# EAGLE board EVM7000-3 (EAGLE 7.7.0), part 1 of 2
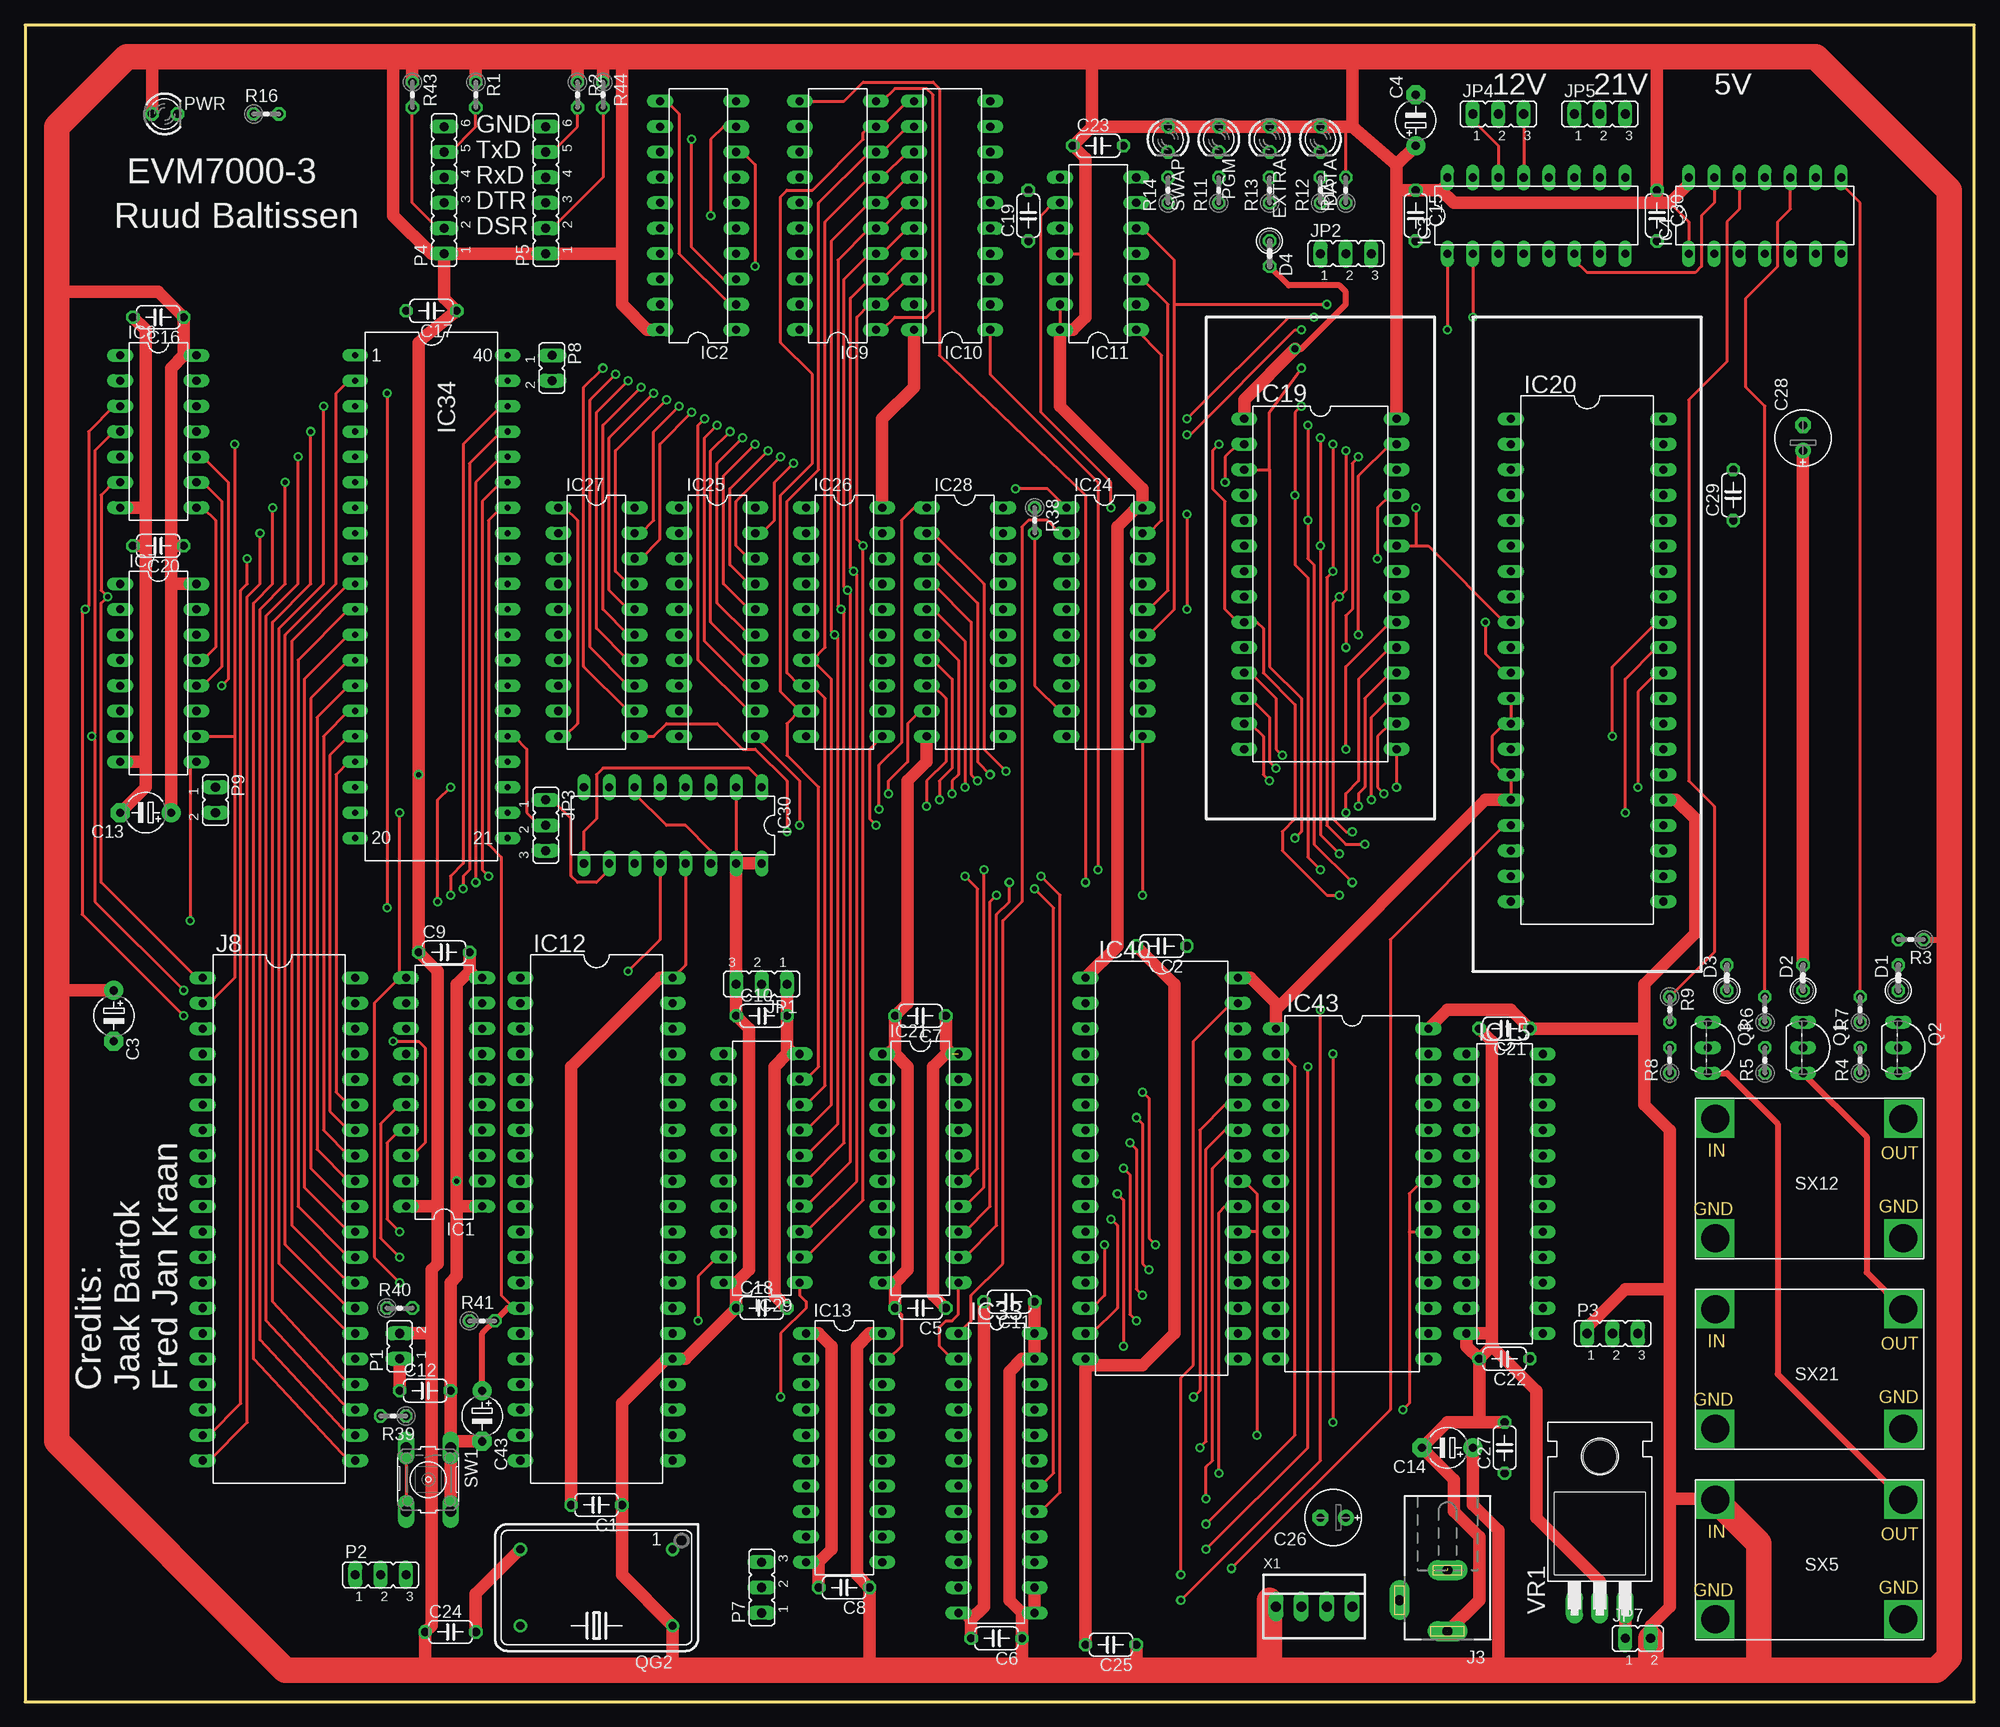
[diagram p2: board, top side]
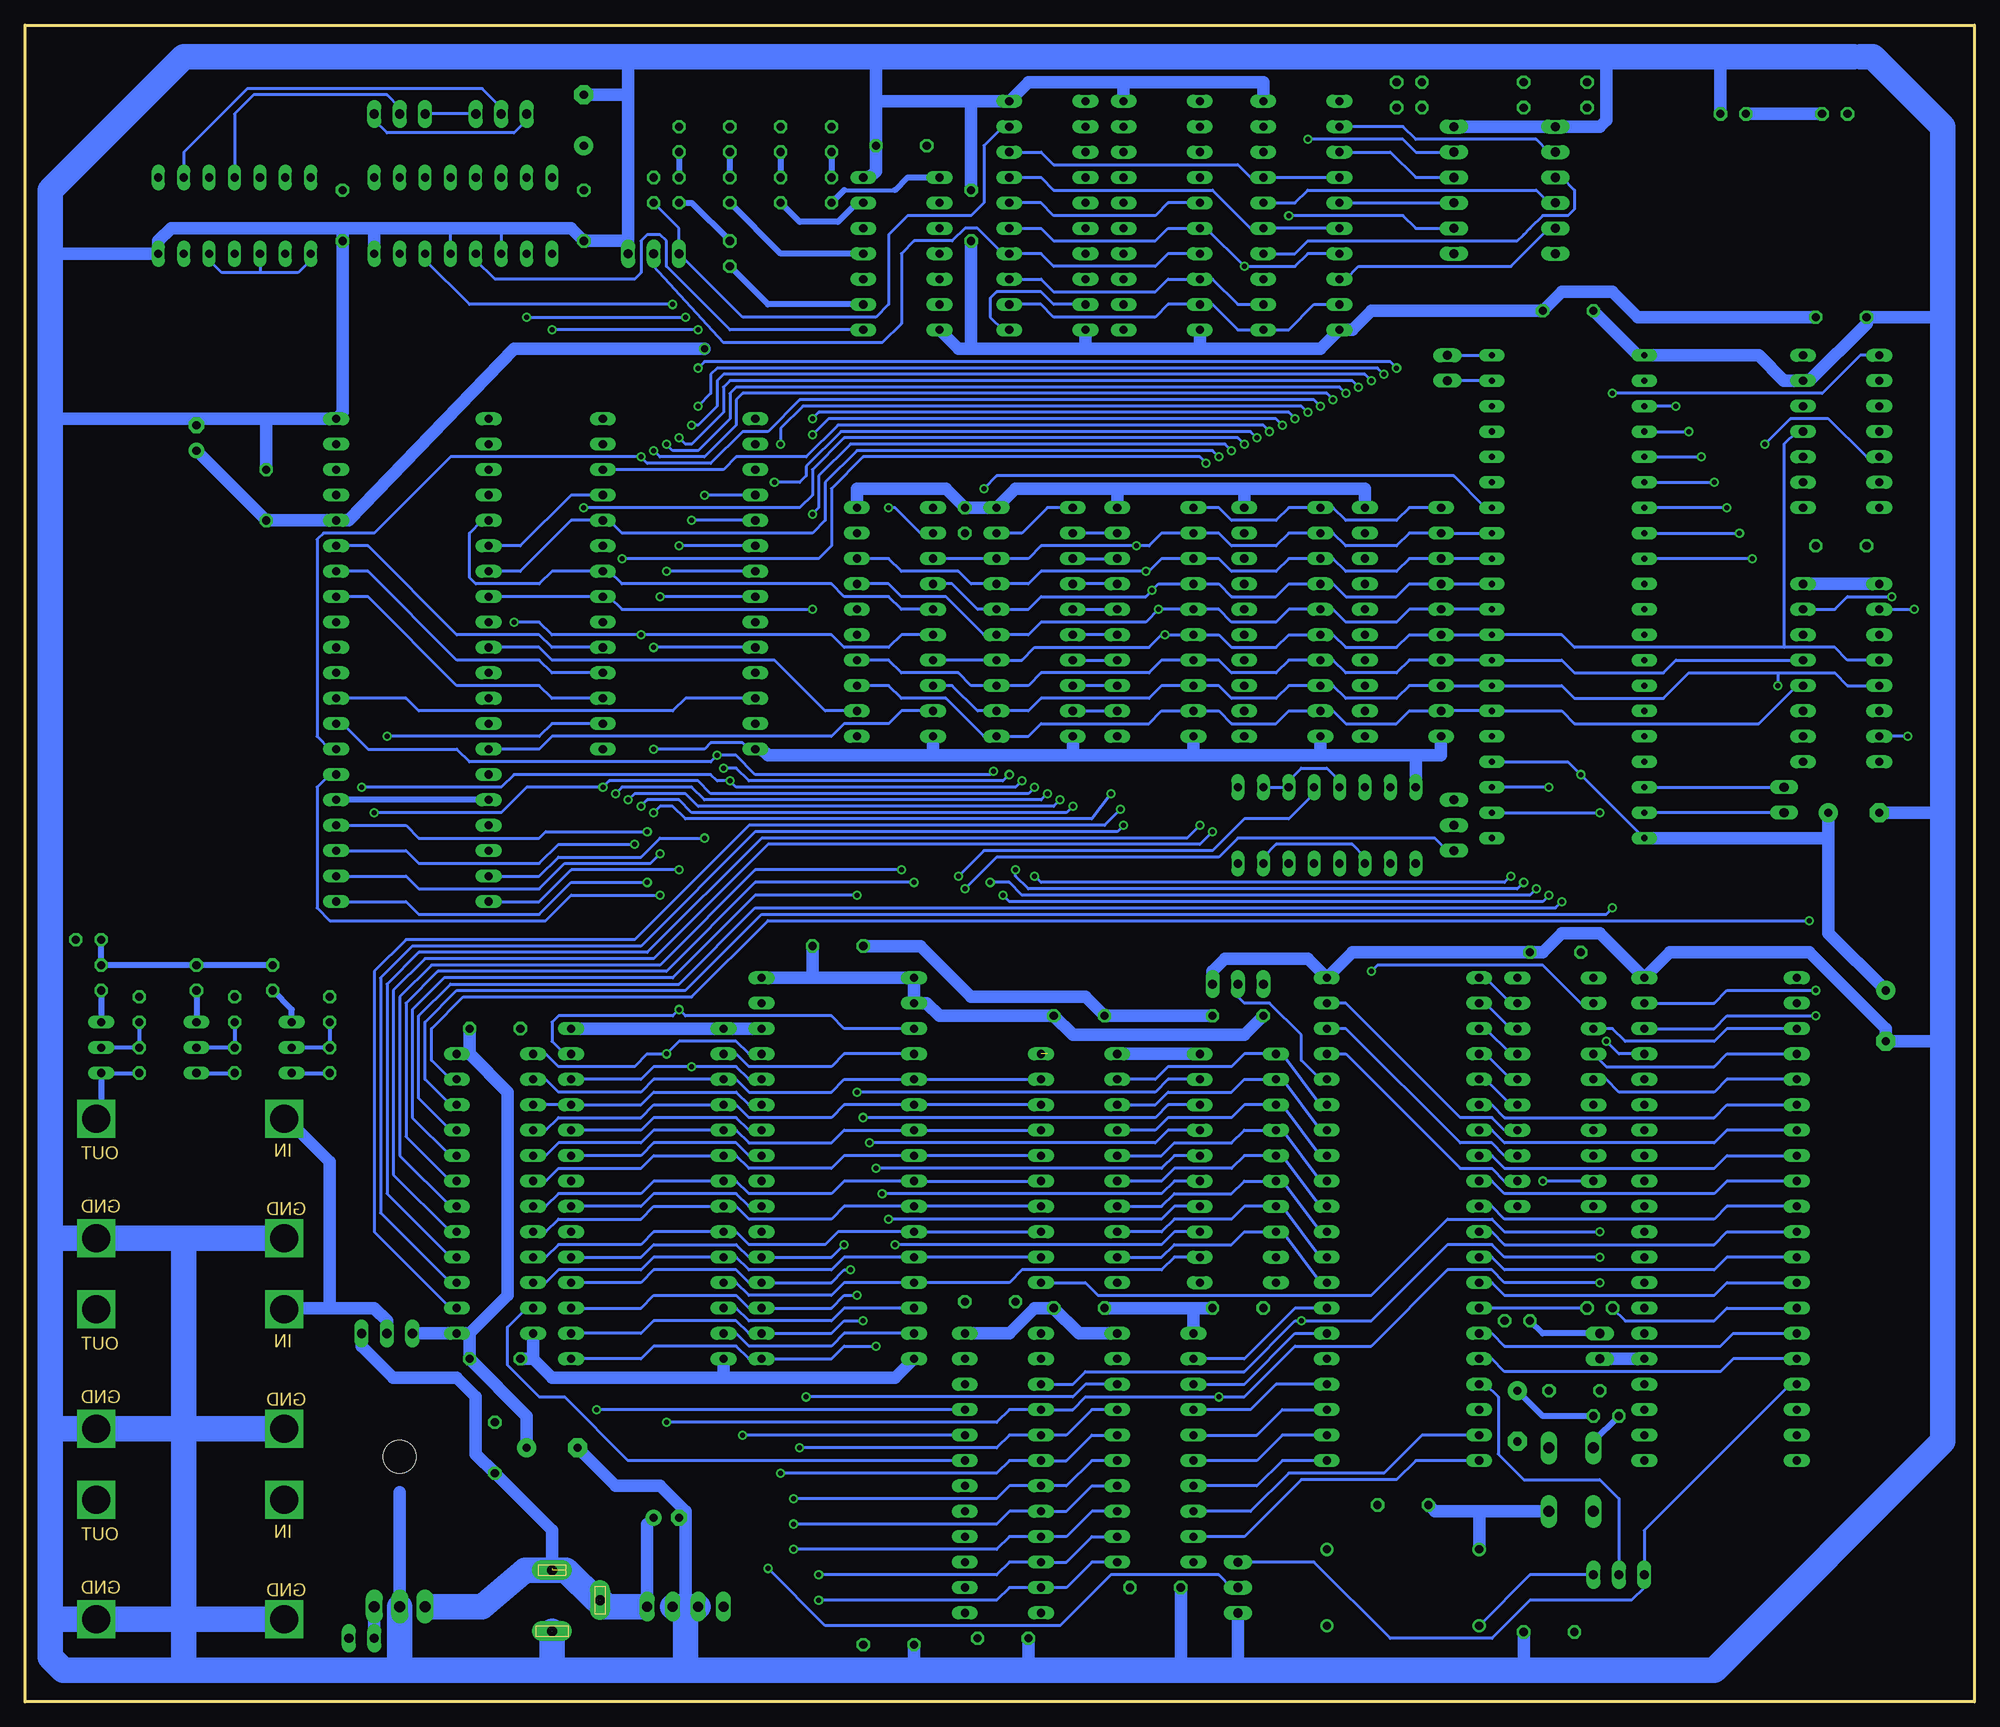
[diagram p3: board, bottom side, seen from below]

Size 194.94 x 167.64 mm. Coordinates in mm from the lower left corner, seen from the top.
Outline: 0,0 194.94,0 194.94,167.64 0,167.64 0,0
Copper layers (1*16): Top 0.035mm / dielectric 1.5mm / Bottom 0.035mm
Design rules "default": minimum track width 10mil, minimum drill 24mil, track to track 8mil, track to pad 8mil, pad to pad 8mil, via to via 8mil, smd to smd 8mil, copper to edge 40mil, drill to drill 8mil, minimum pad ring 10mil, minimum via ring 8mil, stop-mask expansion 4mil, vias tented up to drill 0mil, thermal gap 10mil

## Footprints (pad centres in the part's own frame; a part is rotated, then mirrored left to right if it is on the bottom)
C050-024X044 = drill 0.813 octagon: 1 -2.54,0; 2 2.54,0
E5-4 = drill 0.813 pad 1.905: + -2.54,0 | drill 0.813 pad 1.905 octagon: - 2.54,0
E2,5-6E = drill 0.813 pad 1.575: + -1.27,0 | drill 0.813 pad 1.575 octagon: - 1.27,0
0207/2V = drill 0.813 octagon: 1 -1.27,0; 2 1.27,0
LED3MM = drill 0.813 octagon: A -1.27,0; K 1.27,0
DIL20 = drill 0.813 long: 1 -11.43,-3.81; 2 -8.89,-3.81; 3 -6.35,-3.81; 4 -3.81,-3.81; 5 -1.27,-3.81; 6 1.27,-3.81; 7 3.81,-3.81; 8 6.35,-3.81; 9 8.89,-3.81; 10 11.43,-3.81; 11 11.43,3.81; 12 8.89,3.81; 13 6.35,3.81; 14 3.81,3.81; 15 1.27,3.81; 16 -1.27,3.81; 17 -3.81,3.81; 18 -6.35,3.81; 19 -8.89,3.81; 20 -11.43,3.81
DIL16 = drill 0.813 long: 1 -8.89,-3.81; 2 -6.35,-3.81; 3 -3.81,-3.81; 4 -1.27,-3.81; 5 1.27,-3.81; 6 3.81,-3.81; 7 6.35,-3.81; 8 8.89,-3.81; 9 8.89,3.81; 10 6.35,3.81; 11 3.81,3.81; 12 1.27,3.81; 13 -1.27,3.81; 14 -3.81,3.81; 15 -6.35,3.81; 16 -8.89,3.81
DIL14 = drill 0.813 long: 1 -7.62,-3.81; 2 -5.08,-3.81; 3 -2.54,-3.81; 4 0,-3.81; 5 2.54,-3.81; 6 5.08,-3.81; 7 7.62,-3.81; 8 7.62,3.81; 9 5.08,3.81; 10 2.54,3.81; 11 0,3.81; 12 -2.54,3.81; 13 -5.08,3.81; 14 -7.62,3.81
DIL40 = drill 0.813 long: 1 -24.13,-7.62; 2 -21.59,-7.62; 3 -19.05,-7.62; 4 -16.51,-7.62; 5 -13.97,-7.62; 6 -11.43,-7.62; 7 -8.89,-7.62; 8 -6.35,-7.62; 9 -3.81,-7.62; 10 -1.27,-7.62; 11 1.27,-7.62; 12 3.81,-7.62; 13 6.35,-7.62; 14 8.89,-7.62; 15 11.43,-7.62; 16 13.97,-7.62; 17 16.51,-7.62; 18 19.05,-7.62; 19 21.59,-7.62; 20 24.13,-7.62; 21 24.13,7.62; 22 21.59,7.62; 23 19.05,7.62; 24 16.51,7.62; 25 13.97,7.62; 26 11.43,7.62; 27 8.89,7.62; 28 6.35,7.62; 29 3.81,7.62; 30 1.27,7.62; 31 -1.27,7.62; 32 -3.81,7.62; 33 -6.35,7.62; 34 -8.89,7.62; 35 -11.43,7.62; 36 -13.97,7.62; 37 -16.51,7.62; 38 -19.05,7.62; 39 -21.59,7.62; 40 -24.13,7.62
DIL24-3 = drill 0.813 long: 1 -13.97,-3.81; 2 -11.43,-3.81; 3 -8.89,-3.81; 4 -6.35,-3.81; 5 -3.81,-3.81; 6 -1.27,-3.81; 7 1.27,-3.81; 8 3.81,-3.81; 9 6.35,-3.81; 10 8.89,-3.81; 11 11.43,-3.81; 12 13.97,-3.81; 13 13.97,3.81; 14 11.43,3.81; 15 8.89,3.81; 16 6.35,3.81; 17 3.81,3.81; 18 1.27,3.81; 19 -1.27,3.81; 20 -3.81,3.81; 21 -6.35,3.81; 22 -8.89,3.81; 23 -11.43,3.81; 24 -13.97,3.81
DIL28 = drill 0.813 long: 1 -16.51,-7.62; 2 -13.97,-7.62; 3 -11.43,-7.62; 4 -8.89,-7.62; 5 -6.35,-7.62; 6 -3.81,-7.62; 7 -1.27,-7.62; 8 1.27,-7.62; 9 3.81,-7.62; 10 6.35,-7.62; 11 8.89,-7.62; 12 11.43,-7.62; 13 13.97,-7.62; 14 16.51,-7.62; 15 16.51,7.62; 16 13.97,7.62; 17 11.43,7.62; 18 8.89,7.62; 19 6.35,7.62; 20 3.81,7.62; 21 1.27,7.62; 22 -1.27,7.62; 23 -3.81,7.62; 24 -6.35,7.62; 25 -8.89,7.62; 26 -11.43,7.62; 27 -13.97,7.62; 28 -16.51,7.62
DIP40 = drill 0.61 pad 1.27 long: 1 -24.13,-7.62; 2 -21.59,-7.62; 3 -19.05,-7.62; 4 -16.51,-7.62; 5 -13.97,-7.62; 6 -11.43,-7.62; 7 -8.89,-7.62; 8 -6.35,-7.62; 9 -3.81,-7.62; 10 -1.27,-7.62; 11 1.27,-7.62; 12 3.81,-7.62; 13 6.35,-7.62; 14 8.89,-7.62; 15 11.43,-7.62; 16 13.97,-7.62; 17 16.51,-7.62; 18 19.05,-7.62; 19 21.59,-7.62; 20 24.13,-7.62; 21 24.13,7.62; 22 21.59,7.62; 23 19.05,7.62; 24 16.51,7.62; 25 13.97,7.62; 26 11.43,7.62; 27 8.89,7.62; 28 6.35,7.62; 29 3.81,7.62; 30 1.27,7.62; 31 -1.27,7.62; 32 -3.81,7.62; 33 -6.35,7.62; 34 -8.89,7.62; 35 -11.43,7.62; 36 -13.97,7.62; 37 -16.51,7.62; 38 -19.05,7.62; 39 -21.59,7.62; 40 -24.13,7.62
DIL32-6 = drill 0.813 long: 1 -19.05,-7.62; 2 -16.51,-7.62; 3 -13.97,-7.62; 4 -11.43,-7.62; 5 -8.89,-7.62; 6 -6.35,-7.62; 7 -3.81,-7.62; 8 -1.27,-7.62; 9 1.27,-7.62; 10 3.81,-7.62; 11 6.35,-7.62; 12 8.89,-7.62; 13 11.43,-7.62; 14 13.97,-7.62; 15 16.51,-7.62; 16 19.05,-7.62; 17 19.05,7.62; 18 16.51,7.62; 19 13.97,7.62; 20 11.43,7.62; 21 8.89,7.62; 22 6.35,7.62; 23 3.81,7.62; 24 1.27,7.62; 25 -1.27,7.62; 26 -3.81,7.62; 27 -6.35,7.62; 28 -8.89,7.62; 29 -11.43,7.62; 30 -13.97,7.62; 31 -16.51,7.62; 32 -19.05,7.62
DCJ0202 = drill 1 pad 2 long: 1 0,3.1; 2 4.8,0; 3 0,-3
JP2 = drill 0.914 long: 1 -2.54,0; 2 0,0; 3 2.54,0
JP2P = drill 0.914 long: 1 0,0; 2 2.54,0
JP6E = drill 0.914 long: 1 -3.81,0; 2 -1.27,0; 3 1.27,0; 4 3.81,0; 5 6.35,0; 6 8.89,0
TO92-EBC = drill 0.813 long: B 0,-1.27; C -2.54,-1.27; E 2.54,-1.27
DIL14S = drill 0.813: 1 -7.62,-3.81; 7 7.62,-3.81; 8 7.62,3.81; 14 -7.62,3.81
0204V = drill 0.813 octagon: 1 -1.27,0; 2 1.27,0
B3F-10XX = drill 1.1 long: 1 -3.175,2.223; 2 3.175,2.223; 3 -3.175,-2.223; 4 3.175,-2.223
SX1308 = drill 2.8 square: 1 2.032,13.97; 2 20.828,13.97; 3 20.828,2.032; 4 2.032,2.032
TO220H = drill 1.118 long: 1 -2.54,-10.16; 2 0,-10.16; 3 2.54,-10.16 | hole 3.302: 0,4.826
22-23-2041 = drill 1 long: 1 -3.81,0; 2 -1.27,0; 3 1.27,0; 4 3.81,0

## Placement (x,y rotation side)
C1  100n  [C050-024X044]  57.15,19.68 180 top
C2  100n  [C050-024X044]  113.67,75.56 180 top
C3  10u  [E5-4]  8.89,68.58 270 top
C4  10u  [E5-4]  139.06,158.12 90 top
C5  100n  [C050-024X044]  89.53,39.37 180 top
C6  100n  [C050-024X044]  97.16,6.35 180 top
C7  100n  [C050-024X044]  89.53,68.58 180 top
C8  100n  [C050-024X044]  81.92,11.43 180 top
C9  100n  [C050-024X044]  41.91,74.93 0 top
C10  100n  [C050-024X044]  73.66,68.58 0 top
C11  100n  [C050-024X044]  98.42,40.01 180 top
C12  100n  [C050-024X044]  40.01,31.11 0 top
C13  10u  [E5-4]  12.06,88.9 180 top
C14  10u  [E5-4]  142.24,25.4 180 top
C15  100n  [C050-024X044]  139.06,148.59 270 top
C16  100n  [C050-024X044]  13.34,138.43 180 top
C17  100n  [C050-024X044]  40.64,139.06 180 top
C18  100n  [C050-024X044]  73.66,39.37 0 top
C19  100n  [C050-024X044]  100.33,148.59 90 top
C20  100n  [C050-024X044]  13.34,115.57 180 top
C21  100n  [C050-024X044]  147.96,67.31 180 top
C22  100n  [C050-024X044]  147.96,34.29 180 top
C23  100n  [C050-024X044]  107.31,155.57 0 top
C24  100n  [C050-024X044]  42.55,6.99 0 top
C25  100n  [C050-024X044]  108.58,5.71 180 top
C26  22u  [E2,5-6E]  130.81,18.41 180 top
C27  100n  [C050-024X044]  147.96,25.4 90 top
C28  22u  [E2,5-6E]  177.8,126.36 90 top
C29  100n  [C050-024X044]  170.81,120.65 90 top
C30  100n  [C050-024X044]  163.19,148.59 270 top
C43  4u7  [E5-4]  45.72,28.57 270 top
D1  [0207/2V]  187.32,72.39 90 top
D2  [0207/2V]  177.8,72.39 90 top
D3  [0207/2V]  170.18,72.39 90 top
D4  [0207/2V]  124.46,144.78 270 top
DATA  [LED3MM]  129.54,156.21 270 top
EXTRA  [LED3MM]  124.46,156.21 270 top
IC1  74LS541N  [DIL20]  41.91,60.96 90 top
IC2  74LS241N  [DIL20]  67.31,148.59 90 top
IC3  74LS138N  [DIL16]  151.13,148.59 0 top
IC4  7407N  [DIL14]  173.99,148.59 0 top
IC7  74LS175N  [DIL16]  13.34,102.87 270 top
IC8  74LS243N  [DIL14]  13.34,127 270 top
IC9  74AS574N  [DIL20]  81.28,148.59 90 top
IC10  74LS541N  [DIL20]  92.71,148.59 90 top
IC11  74LS06N  [DIL14]  107.31,144.78 90 top
IC12  TMS7000  [DIL40]  57.15,48.26 270 top
IC13  74LS541N  [DIL20]  81.92,25.4 270 top
IC15  GAL22V10  [DIL24-3]  147.96,50.8 270 top
IC19  27256OUT  [DIL28]  129.54,111.76 270 top
IC20  TMS7000-Contra  [DIL40]  156.21,104.14 270 top
IC21  74AS573N  [DIL20]  89.53,53.34 270 top
IC24  74LS273N  [DIL20]  107.95,107.95 270 top
IC25  74AS574N  [DIL20]  69.22,107.95 270 top
IC26  74AS574N  [DIL20]  81.92,107.95 270 top
IC27  74AS574N  [DIL20]  57.15,107.95 270 top
IC28  74LS541N  [DIL20]  93.98,107.95 270 top
IC29  74LS245N  [DIL20]  73.66,53.34 90 top
IC30  74LS109N  [DIL16]  64.77,87.63 180 top
IC33  GAL20V8  [DIL24-3]  97.16,22.86 270 top
IC34  6522  [DIP40]  40.64,110.49 270 top
IC40  681000  [DIL32-6]  113.67,53.34 270 top
IC43  27256  [DIL28]  132.72,50.8 270 top
J3  DCJ0202  [DCJ0202]  142.24,10.16 180 top
J8  TMS7000-Contra  [DIL40]  25.4,48.26 270 top
JP1  [JP2]  73.66,71.75 180 top
JP2  [JP2]  132.08,144.78 0 top
JP3  [JP2]  52.07,87.63 270 top
JP4  [JP2]  147.32,158.75 0 top
JP5  [JP2]  157.48,158.75 0 top
JP7  [JP2P]  160.02,6.35 0 top
P1  JP2P  [JP2P]  37.47,34.29 90 top
P2  [JP2]  35.56,12.7 0 top
P3  [JP2]  158.75,36.83 0 top
P4  JP6E  [JP6E]  41.91,148.59 90 top
P5  JP6E  [JP6E]  52.07,148.59 90 top
P7  [JP2]  73.66,11.43 90 top
P8  JP2P  [JP2P]  52.7,134.62 270 top
P9  JP2P  [JP2P]  19.05,91.44 270 top
PGM  [LED3MM]  119.38,156.21 270 top
PWR  [LED3MM]  13.97,158.75 0 top
Q1  BC557  [TO92-EBC]  179.07,65.41 270 top
Q2  BC557  [TO92-EBC]  188.59,65.41 270 top
Q3  BC557  [TO92-EBC]  169.54,65.41 270 top
QG2  4 MHz  [DIL14S]  57.15,11.43 180 top
R1  1K  [0204V]  45.09,160.66 270 top
R2  1K  [0204V]  55.24,160.66 270 top
R3  1K  [0204V]  188.59,76.2 180 top
R4  1K  [0204V]  183.51,64.14 90 top
R5  1K  [0204V]  173.99,64.14 90 top
R6  1K  [0204V]  173.99,69.22 90 top
R7  1K  [0204V]  183.51,69.22 90 top
R8  1K  [0204V]  164.47,64.14 90 top
R9  1K  [0204V]  164.47,69.22 270 top
R11  1K  [0204V]  119.38,151.13 90 top
R12  1K  [0204V]  129.54,151.13 90 top
R13  1K  [0204V]  124.46,151.13 90 top
R14  1K  [0204V]  114.3,151.13 90 top
R15  1K  [0204V]  132.08,151.13 90 top
R16  1K  [0204V]  24.13,158.75 0 top
R38  1K  [0204V]  100.97,118.11 270 top
R39  22  [0204V]  36.83,28.57 180 top
R40  47  [0204V]  37.47,39.37 0 top
R41  2K2  [0204V]  45.72,38.1 0 top
R43  1K  [0204V]  38.73,160.66 270 top
R44  1K  [0204V]  57.78,160.66 270 top
SW1  [B3F-10XX]  40.32,22.23 270 top
SWAP  [LED3MM]  114.3,156.21 270 top
SX5  SX1308  [SX1308]  189.87,22.23 180 top
SX12  SX1308  [SX1308]  189.87,60.33 180 top
SX21  SX1308  [SX1308]  189.87,41.27 180 top
VR1  7805T  [TO220H]  157.48,19.68 0 top
X1  PC-Power  [22-23-2041]  128.91,9.53 0 top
